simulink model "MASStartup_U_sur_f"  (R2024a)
settings: Solver=FixedStepAuto  StartTime=0.0  StopTime=2  FixedStep=Ts  RelTol=1e-3  AbsTol=1e-3  EnableMultiTasking=on
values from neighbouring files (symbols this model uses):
  Tn = Pn/(Nn*2*pi/60)    (= 14.6912255162)    [ConstantsMAS_U_sur_f.m]
  Ts = 5e-6    (= 5e-06)    [ConstantsMAS_U_sur_f.m]
libraries: nesl_utility x8, ee_lib x2, eePwmGeneratorTwoLevel x1, eeGeneralControl x1

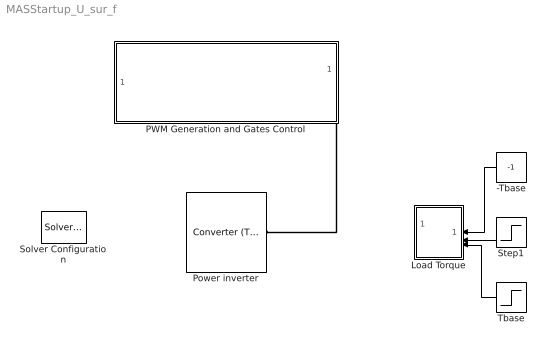
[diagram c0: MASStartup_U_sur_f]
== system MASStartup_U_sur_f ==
  -Tbase : Constant  Value=-1  SampleTime=0
  Load Torque : Subsystem
  PWM Generation and Gates Control : Subsystem
  Power inverter : ee_lib/Semiconductors & Converters/Converters/Converter (Three-Phase)  port_option=ee.enum.threePhasePort.composite  fidelity_option=ee.enum.converters.fidelity.detailed  device_type=3  K=0  Vf=0.8 V  Ron=0.001 Ohm  Rds=0.001 Ohm  Goff=1e-5 1/Ohm  Vgt=1 V  Vgt_off=-1 V  Ih=1 A  Vth=0.5 V  diode_param=2  diode_Vf=0.8 V  diode_Ron=0.001 Ohm  diode_Goff=1e-5 1/Ohm  diode_C=50 nF  diode_iRM=-235 A  diode_iF=300 A  diode_idot=-50 A/us  diode_trr_param=1  diode_trr_factor=3  diode_trr=15 us  diode_Qrr=1.5e+3 s*uA  snubber_type=0  Cs=1e-7 F  Rs=0.1 Ohm
  Solver Configuration : nesl_utility/Solver Configuration  PhysicalDomain=network_engine_domain  SubClassName=solver  LeftPortType=input  RightPortType=generic  Tones=[]  Harmonics=[]  SimulateNoise=off  Profile=off  UseLocalSampling=off  EnableSwitchedLinearOptims=on  FrequencyDomain=off  UseCCode=off  RelTol=0.001  AbsTol=1e-06  MinStep=1e-09  ToWorkspace=off  RevertToSquareIcSolve=off  NumHomotopyIterations=100  PhasorMode=off  PhasorModeNumHarmonics=1  ConsistencySolver=NEWTON_FTOL  IndexReductionMethod=DerivativeReplacement  DoDC=off  ResidualTolerance=1e-09  ConsistencyTolSource=GLOBAL  ConsistencyAbsTol=0.001  ConsistencyRelTol=0.001  ConsistencyTolFactor=0.001  UseLocalSolver=on  LocalSolverChoice=NE_BACKWARD_EULER_ADVANCER  ResolveIndetEquations=on  FunctionEvalNumThread=1  LocalSolverSampleTime=Ts  DoFixedCost=on  MaxNonlinIter=5  MaxModeIter=2  ComputeImpulses=off  ImpulseIterations=2  LinearAlgebra=auto  LinearAlgebraNumThread=0  EquationFormulation=NE_TIME_EF  DelaysMemoryBudget=1024  AutomaticFiltering=on  FilteringTimeConstant=0.001  PartitionStorageMethod=AS_NEEDED  PartitionMemoryBudget=1024  PartitionMethod=ROBUST  MultibodyUseLocalSolver=off  MultibodyLocalSolverChoice=ODE1  MultibodyLocalSolverSampleTime=0.001
  Step1 : Step  Time=1.5  SampleTime=0
  Tbase : Step  SampleTime=0
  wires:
  Tbase/1 -> Load Torque/3(Tn)
  -Tbase/1 -> Load Torque/1(-Tn)
  Step1/1 -> Load Torque/2(Step)
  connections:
  Power inverter/LConn1 -- PWM Generation and Gates Control/RConn1

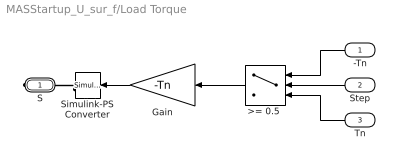
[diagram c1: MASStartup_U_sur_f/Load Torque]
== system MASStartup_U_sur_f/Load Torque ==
  -Tn : Inport
  Step : Inport  Port=2
  Tn : Inport  Port=3
  ">= 0.5 " : Switch  Threshold=0.5
  Gain : Gain  Gain=-Tn
  Simulink-PS Converter : nesl_utility/Simulink-PS Converter  PhysicalDomain=network_engine_domain  SubClassName=ps_input  LeftPortType=input  RightPortType=output  PseudoPeriodic=off  Frequencies=[]  NoiseDistribution=none  NoiseParameters=[]  Unit=1  AffineConversion=off  FilteringAndDerivatives=zero  SimscapeFilterOrder=1  InputFilterTimeConstant=0.001  UdotUserProvided=1
  S : PMIOPort  Side=Right
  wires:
  ">= 0.5 "/1 -> Gain/1
  -Tn/1 -> ">= 0.5 "/1
  Step/1 -> ">= 0.5 "/2
  Gain/1 -> Simulink-PS Converter/1
  Tn/1 -> ">= 0.5 "/3
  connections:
  Simulink-PS Converter/RConn1 -- S/RConn1

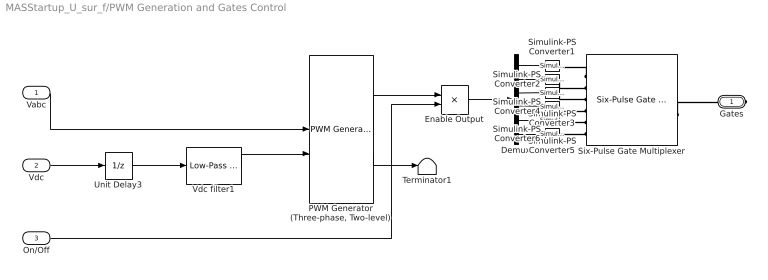
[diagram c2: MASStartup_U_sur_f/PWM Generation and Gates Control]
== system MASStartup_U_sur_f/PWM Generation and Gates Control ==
  Vabc : Inport
  Vdc : Inport  Port=2
  On/Off : Inport  Port=3
  Demux : Demux  Outputs=6
  Enable Output : Product
  "PWM Generator (Three-phase, Two-level)" : eePwmGeneratorTwoLevel/PWM Generator (Three-phase, Two-level)  PWMMode=Continuous PWM (CPWM)  CPWMMode=SPWM: sinusoidal PWM  DPWMMode=60 DPWM: 60 degree discontinuous PWM  fsw=fsw  Ts=Ts
  Simulink-PS Converter{1..6} (6 alike) : nesl_utility/Simulink-PS Converter  PhysicalDomain=network_engine_domain  SubClassName=ps_input  LeftPortType=input  RightPortType=output  PseudoPeriodic=off  Frequencies=[]  NoiseDistribution=none  NoiseParameters=[]  Unit=1  AffineConversion=off  FilteringAndDerivatives=zero  SimscapeFilterOrder=1  InputFilterTimeConstant=0.001  UdotUserProvided=1
  Six-Pulse Gate Multiplexer : ee_lib/Semiconductors & Converters/Converters/Six-Pulse Gate Multiplexer  port_option=ee.enum.controlport.ps
  Terminator1 : Terminator
  Unit Delay3 : UnitDelay  SampleTime=-1  HasFrameUpgradeWarning=on
  Vdc filter1 : eeGeneralControl/Low-Pass Filter (Discrete or Continuous)  K=1  T=1e-3  B=inf  A=-inf  init_option=Inherited from block input  x0=0  Ts=-1
  Gates : PMIOPort  Side=Right
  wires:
  Unit Delay3/1 -> Vdc filter1/1
  "PWM Generator (Three-phase, Two-level)"/2 -> Terminator1/1
  "PWM Generator (Three-phase, Two-level)"/1 -> Enable Output/1
  Vabc/1 -> "PWM Generator (Three-phase, Two-level)"/1
  Demux/2 -> Simulink-PS Converter2/1
  Enable Output/1 -> Demux/1
  Demux/3 -> Simulink-PS Converter3/1
  Demux/5 -> Simulink-PS Converter5/1
  Demux/6 -> Simulink-PS Converter6/1
  Demux/4 -> Simulink-PS Converter4/1
  Demux/1 -> Simulink-PS Converter1/1
  On/Off/1 -> Enable Output/2
  Vdc/1 -> Unit Delay3/1
  Vdc filter1/1 -> "PWM Generator (Three-phase, Two-level)"/2
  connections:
  Simulink-PS Converter4/RConn1 -- Six-Pulse Gate Multiplexer/LConn4
  Six-Pulse Gate Multiplexer/LConn1 -- Simulink-PS Converter1/RConn1
  Simulink-PS Converter3/RConn1 -- Six-Pulse Gate Multiplexer/LConn3
  Simulink-PS Converter6/RConn1 -- Six-Pulse Gate Multiplexer/LConn6
  Simulink-PS Converter2/RConn1 -- Six-Pulse Gate Multiplexer/LConn2
  Six-Pulse Gate Multiplexer/RConn1 -- Gates/RConn1
  Simulink-PS Converter5/RConn1 -- Six-Pulse Gate Multiplexer/LConn5
